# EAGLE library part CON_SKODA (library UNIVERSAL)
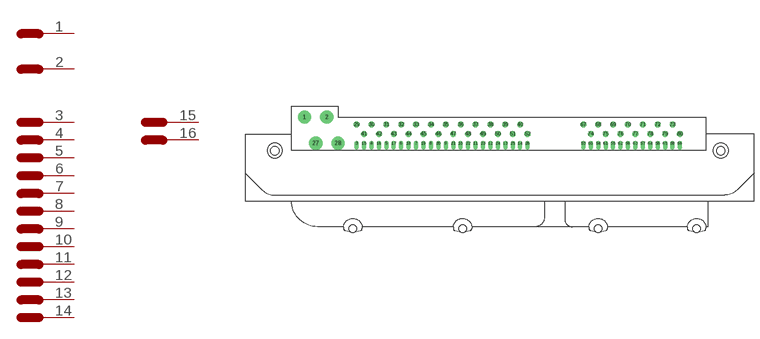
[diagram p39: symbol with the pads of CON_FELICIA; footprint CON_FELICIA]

Designator prefix CON; gates 1=PIN 2=PIN 3=PIN 4=PIN 5=PIN 6=PIN 7=PIN 8=PIN 9=PIN 10=PIN 11=PIN 12=PIN 13=PIN 14=PIN 15=PIN 16=PIN 17=PIN 18=PIN 19=PIN 20=PIN 21=PIN 22=PIN 23=PIN 24=PIN 25=PIN 26=PIN 27=PIN 28=PIN 29=PIN 30=PIN 31=PIN 32=PIN 33=PIN 34=PIN 35=PIN 36=PIN 37=PIN 38=PIN 39=PIN 40=PIN 41=PIN 42=PIN 43=PIN 44=PIN 45=PIN 46=PIN 47=PIN 48=PIN 49=PIN 50=PIN 51=PIN 52=PIN 53=PIN 54=PIN 55=PIN 56=PIN 57=PIN 58=PIN 59=PIN 60=PIN 61=PIN 62=PIN 63=PIN 64=PIN 65=PIN 66=PIN 67=PIN 68=PIN 69=PIN 70=PIN 71=PIN 72=PIN 73=PIN 74=PIN 75=PIN 76=PIN 77=PIN 78=PIN 79=PIN 80=PIN

## CON_SKODA  [CON_FELICIA]
1  1:1
2  2:1
3  3:1
4  4:1
5  5:1
6  6:1
7  7:1
8  8:1
9  9:1
10  10:1
11  11:1
12  12:1
13  13:1
14  14:1
15  15:1
16  16:1
17  17:1
18  18:1
19  19:1
20  20:1
21  21:1
22  22:1
23  23:1
24  24:1
25  25:1
26  26:1
27  27:1
28  28:1
29  29:1
30  30:1
31  31:1
32  32:1
33  33:1
34  34:1
35  35:1
36  36:1
37  37:1
38  38:1
39  39:1
40  40:1
41  41:1
42  42:1
43  43:1
44  44:1
45  45:1
46  46:1
47  47:1
48  48:1
49  49:1
50  50:1
51  51:1
52  52:1
53  53:1
54  54:1
55  55:1
56  56:1
57  57:1
58  58:1
59  59:1
60  60:1
61  61:1
62  62:1
63  63:1
64  64:1
65  65:1
66  66:1
67  67:1
68  68:1
69  69:1
70  70:1
71  71:1
72  72:1
73  73:1
74  74:1
75  75:1
76  76:1
77  77:1
78  78:1
79  79:1
80  80:1

## Footprint CON_FELICIA (pad centres in mm)
drill 0.7 pad 3.81: 1 -14.98,7.49; 2 -8.56,7.49
drill 0.8 pad 1.27 offset: 3 0,0; 4 4.28,0; 5 8.56,0; 6 12.84,0; 7 17.12,0; 8 21.4,0; 9 25.68,0; 10 29.96,0; 11 34.24,0; 12 38.52,0; 13 42.8,0; 14 47.08,0; 15 2.14,0; 16 6.42,0; 17 10.7,0; 18 14.98,0; 19 19.26,0; 20 23.54,0; 21 27.82,0; 22 32.1,0; 23 36.38,0; 24 40.66,0; 25 44.94,0; 26 49.22,0; 53 65.27,0; 54 69.55,0; 55 73.83,0; 56 78.11,0; 57 82.39,0; 58 86.67,0; 59 90.95,0; 60 67.41,0; 61 71.69,0; 62 75.97,0; 63 80.25,0; 64 84.53,0; 65 88.81,0; 66 93.09,0
drill 0.8 pad 3.81: 27 -11.77,0; 28 -5.35,0
drill 0.7 pad 1.676: 29 0,5.35; 30 4.28,5.35; 31 8.56,5.35; 32 12.84,5.35; 33 17.12,5.35; 34 21.4,5.35; 35 25.68,5.35; 36 29.96,5.35; 37 34.24,5.35; 38 38.52,5.35; 39 42.8,5.35; 40 47.08,5.35; 41 2.14,2.675; 42 6.42,2.675; 43 10.7,2.675; 44 14.98,2.675; 45 19.26,2.675; 46 23.54,2.675; 47 27.82,2.675; 48 32.1,2.675; 49 36.38,2.675; 50 40.66,2.675; 51 44.94,2.675; 52 49.22,2.675; 67 65.27,5.35; 68 69.55,5.35; 69 73.83,5.35; 70 78.11,5.35; 71 82.39,5.35; 72 86.67,5.35; 73 90.95,5.35; 74 67.41,2.675; 75 71.69,2.675; 76 75.97,2.675; 77 80.25,2.675; 78 84.53,2.675; 79 88.81,2.675; 80 93.09,2.675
